PROGRAM BEDROOM
VAR	
	fbLight1: FB_Light;
	fbLight2: FB_Light;
	
	R_TRIG_BlindUp: R_TRIG;	
	R_TRIG_BlindDown: R_TRIG;
	bSwitchBlindUp: BOOL;
	bSwitchBlindDown: BOOL;
	fbVenetianBlind: FB_VenetianBlind;	
END_VAR

// Light 1
fbLight1(bOn:= , bOff:= , bToggle:= GVL.I_bTerm2_Var9, bLight=> GVL.Q_bTerm4_Var1);

// Light 2
fbLight2(bOn:= , bOff:= , bToggle:= GVL.I_bTerm2_Var10, bLight=> GVL.Q_bTerm4_Var2);
		
// Blind 1
R_TRIG_BlindUp(CLK:=GVL.I_bTerm2_Var11);
bSwitchBlindUp:=R_TRIG_BlindUp.Q;
R_TRIG_BlindDown(CLK:=GVL.I_bTerm2_Var12);
bSwitchBlindDown:= R_TRIG_BlindDown.Q;

fbVenetianBlind(
	bUp:= bSwitchBlindUp, 
	bDown:= bSwitchBlindDown, 
	bStop:= (bSwitchBlindUp OR bSwitchBlindDown) AND (fbVenetianBlind.bBlindUp OR fbVenetianBlind.bBlindDown), 
	bSwitchOverUp:= , 
	bSwitchOverDown:= , 
	tSwitchOverTime:= , 
	bStepUp:= , 
	bStepDown:= , 
	tStepTime:= , 
	bShadowPosition:= , 
	tShadowTurnAroundTime:= , 
	tShadowTurnOffTime:= , 
	bSafetyPosition:= , 
	tTurnOffTime:= , 
	tSwitchOverDeadTime:= , 
	bBlindUp=> GVL.Q_bTerm11_Var1, 
	bBlindDown=> GVL.Q_bTerm11_Var2);

END_PROGRAM
